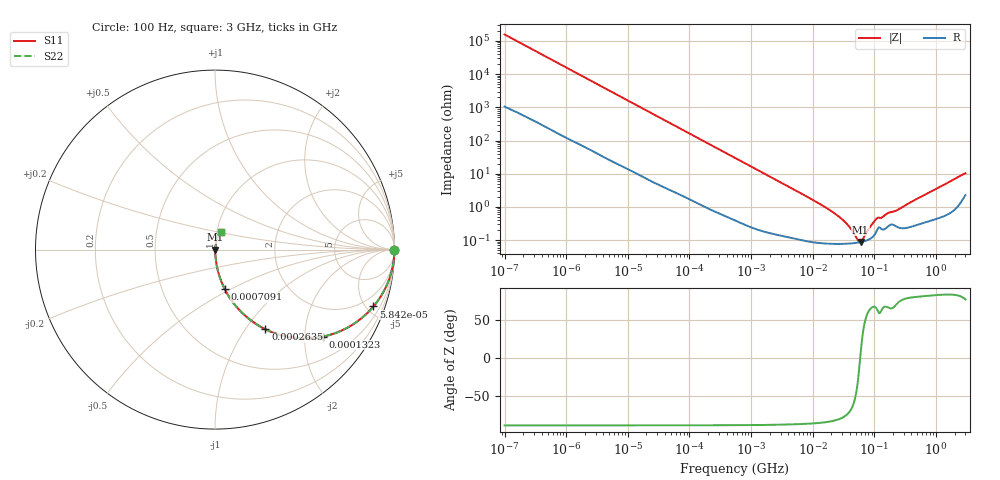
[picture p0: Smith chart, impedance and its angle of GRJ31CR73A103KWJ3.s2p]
!Murata Part Number: GRJ31CR73A103KWJ3
!These Parameters are Measured in Series Mode Connection
!Data Generated on Jun 19, 2026
!  o--ll--o
!Port1  Port2
!  o------o
!Operation Temp=25[degC], DC Bias Voltage=0[V]
!Freq. Start=100[Hz] Stop=3[GHz] 401[Steps]
# Hz S RI R 50
!Freq.(Hz) S11(Real) S11(Imag) S21(Real) S21(Imag) S12(Real) S12(Imag) S22(Real) S22(Imag)
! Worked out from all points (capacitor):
!   401 points, 100 Hz to 3 GHz, reference 50 ohm
!   read as one part in series: C = 10.1 nF near 109 Hz
!   lowest |Z| = 87.5 mohm at 59.71 MHz (marker M1)
!   series resonance near 58.95 MHz, so ESL is about 720 pH
!   S11 on the Smith chart (normalised r, x): 100 Hz: open; 58.42 kHz: 1.06, -5.55; 132.3 kHz: 1.03, -2.46; 263.5 kHz: 1.01, -1.24; 709.1 kHz: 1.01, -0.46; 3 GHz: 1.05, +0.20
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100  1 -0.000638  4.7e-06 0.000638  4.7e-06 0.000638  1 -0.000638
1788  0.9998 -0.0112  0.000216 0.0112  0.000216 0.0112  0.9998 -0.0112
10003  0.9956 -0.062  0.0044 0.062  0.0044 0.062  0.9956 -0.062
31977  0.9607 -0.1899  0.0393 0.1899  0.0393 0.1899  0.9607 -0.1899
58416  0.8826 -0.317  0.1174 0.317  0.1174 0.317  0.8826 -0.317
86054  0.7786 -0.41  0.2214 0.41  0.2214 0.41  0.7786 -0.41
132342  0.6016 -0.4843  0.3984 0.4843  0.3984 0.4843  0.6016 -0.4843
263501  0.2806 -0.4436  0.7194 0.4436  0.7194 0.4436  0.2806 -0.4436
547723  0.0857 -0.2735  0.9143 0.2735  0.9143 0.2735  0.0857 -0.2735
709116  0.0539 -0.2192  0.9461 0.2192  0.9461 0.2192  0.0539 -0.2192
2079876  0.00787 -0.0789  0.9921 0.0789  0.9921 0.0789  0.00787 -0.0789
9794414  0.00115 -0.0167  0.9988 0.0167  0.9988 0.0167  0.00115 -0.0167
2.872754e7  0.000791 -0.00449  0.9992 0.00449  0.9992 0.00449  0.000791 -0.00449
3.882828e7  0.000795 -0.00247  0.9992 0.00247  0.9992 0.00247  0.000795 -0.00247
5.478864e7  0.000846 -0.000425  0.9992 0.000425  0.9992 0.000425  0.000846 -0.000425
5.9714e7  0.000871 7.58e-05  0.9991 -7.58e-05  0.9991 -7.58e-05  0.000871 7.58e-05
6.508213e7  0.000903 0.000581  0.9991 -0.000581  0.9991 -0.000581  0.000903 0.000581
8.425944e7  0.00108 0.00219  0.9989 -0.00219  0.9989 -0.00219  0.00108 0.00219
1.044919e8  0.00163 0.00376  0.9984 -0.00376  0.9984 -0.00376  0.00163 0.00376
1.751444e8  0.00282 0.00619  0.9972 -0.00619  0.9972 -0.00619  0.00282 0.00619
2.36726e8  0.00254 0.00765  0.9975 -0.00765  0.9975 -0.00765  0.00254 0.00765
3e9  0.0317 0.0953  0.9683 -0.0953  0.9683 -0.0953  0.0317 0.0953
